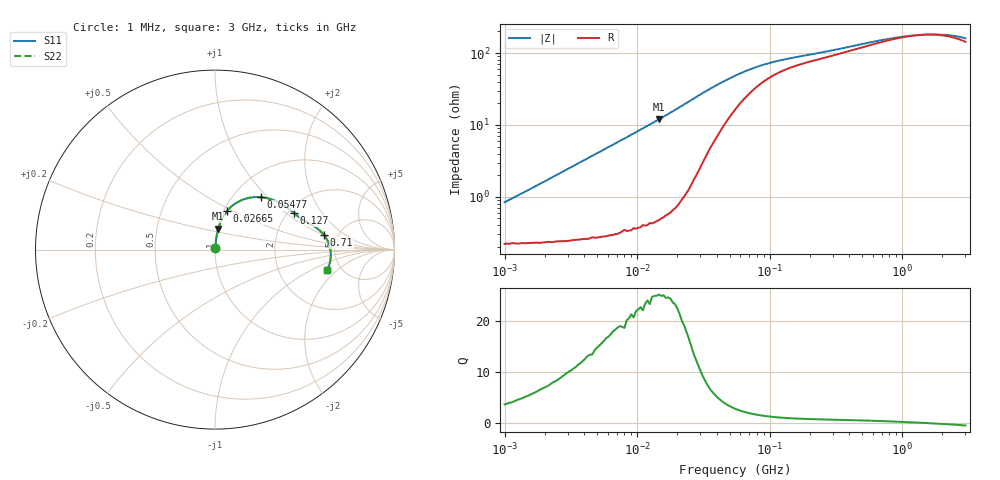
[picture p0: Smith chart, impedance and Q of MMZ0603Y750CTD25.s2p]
! S-Parameter Data Generated by TDK Corporation
! Copyright(C) 2025 TDK Corporation.
! All Rights Reserved.
! TDK P/N: MMZ0603Y750CTD25 (Chip Bead)
! Property: |Z|=75ohm at 100MHz
! Size(LxWxT): 0.6x0.3x0.3mm
! Model Type: s2p (Touchstone File Format Version 1.0)
! Frequency: DC=Yes Start=1MHz Stop=3000MHz 202points Log-sweep
! Model Generated on Feb. 6, 2025
! Terms and conditions regarding TDK Simulation Models:
! 1)This simulation model is being provided solely for informational
!  purposes. Please refer to the specifications of the products in
!  terms of detailed characteristics of such products.
! 2)In no event shall TDK Corporation of any of its subsidiaries be
!  liable for any loss or damage arising, directly or indirectly,
!  from any information contained in this simulation model, including,
!  but not limited to loss or damages arising from any inaccuracies,
!  omissions or errors in connection with such information.
! 3)Any and all copyrights on this simulation model are owned by
!  TDK Corporation.  Duplication or redistribution of this simulation
!  model without prior written permission from TDK Corporation
!  is prohibited.
! 4)This simulation model is subject to any modification or change
!  without any prior notice.
! 5)Neither TDK Corporation nor any of its subsidiaries shall make any
!  warranty, express or implied, including but not limited to the
!  correctness, implied warranties of merchantability and fitness for
!  a particular purpose with respect to this simulation models.
! 6)The use of this simulation model shall be deemed to have consented
!  to the terms and conditions hereof.
! Port Assignments:
!  1 ---@@@--- 2
! Applicable Conditions:
!  Temperature = 25 degC
!  DC Bias Current = 0 A
!  Small Signal Operation
# Hz S MA R 50
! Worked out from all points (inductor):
!   201 points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, 1 MHz to 3 GHz, reference 50 ohm
!   read as one part in series: L = 129 nH near 1.041 MHz
!   highest Q = 25 at 14.62 MHz (marker M1), where L = 130 nH
!   self-resonance near 1.448 GHz
!   S11 on the Smith chart (normalised r, x): 1 MHz: 1.00, +0.02; 26.65 MHz: 1.03, +0.46; 54.77 MHz: 1.33, +0.91; 127 MHz: 2.15, +1.15; 710 MHz: 3.87, +1.02; 3 GHz: 3.87, -1.44
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1000000  0.008403 74.2  0.9977 -0.5  0.9977 -0.5  0.008403 74.2
3900413  0.03154 83.5  0.9969 -1.8  0.9969 -1.8  0.03154 83.5
8686058  0.06972 83.2  0.9942 -4.0  0.9942 -4.0  0.06972 83.2
1.461624e7  0.1185 80.9  0.9883 -6.8  0.9883 -6.8  0.1185 80.9
2.013356e7  0.1658 77.9  0.9788 -9.5  0.9788 -9.5  0.1658 77.9
2.664524e7  0.2228 73.0  0.9587 -12.8  0.9587 -12.8  0.2228 73.0
3.127247e7  0.261 68.8  0.9377 -15.0  0.9377 -15.0  0.261 68.8
3.820236e7  0.309 62.3  0.899 -17.7  0.899 -17.7  0.309 62.3
4.483659e7  0.3463 56.5  0.8587 -19.6  0.8587 -19.6  0.3463 56.5
5.477226e7  0.3876 48.9  0.8006 -21.4  0.8006 -21.4  0.3876 48.9
6.690963e7  0.4211 41.7  0.7405 -22.2  0.7405 -22.2  0.4211 41.7
8.507507e7  0.4514 34.1  0.6754 -22.0  0.6754 -22.0  0.4514 34.1
1.039275e8  0.4697 29.0  0.6318 -21.1  0.6318 -21.1  0.4697 29.0
1.269575e8  0.4843 25.0  0.5972 -20.0  0.5972 -20.0  0.4843 25.0
2.136344e8  0.5185 18.3  0.5332 -17.8  0.5332 -17.8  0.5185 18.3
4.219165e8  0.5733 12.6  0.458 -15.9  0.458 -15.9  0.5733 12.6
7.099691e8  0.6122 7.7  0.4018 -11.8  0.4018 -11.8  0.6122 7.7
8.005644e8  0.6195 6.5  0.3907 -10.3  0.3907 -10.3  0.6195 6.5
1.194682e9  0.6378 2.2  0.3635 -3.9  0.3635 -3.9  0.6378 2.2
1.712864e9  0.6457 -2.1  0.3555 3.7  0.3555 3.7  0.6457 -2.1
2.266846e9  0.6451 -5.8  0.364 10.3  0.364 10.3  0.6451 -5.8
3e9  0.6325 -10.2  0.3938 16.5  0.3938 16.5  0.6325 -10.2
